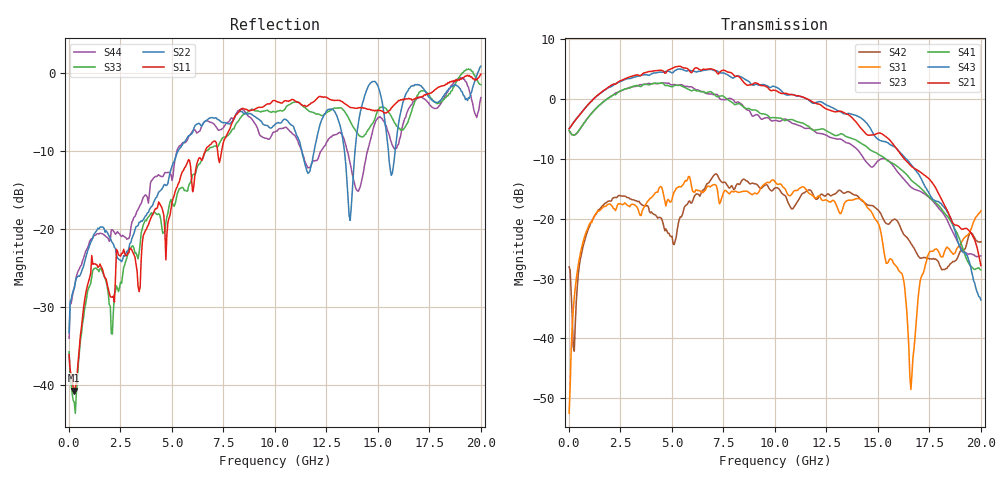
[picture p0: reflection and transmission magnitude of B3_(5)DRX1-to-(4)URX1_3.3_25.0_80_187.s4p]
!Agilent Technologies,N5225A,MY51451112,A.09.50.13
!Agilent N5225A: A.09.50.13
!Date: Sunday, March 12, 2017 05:22:41
!Correction: S11(Full 4 Port(1,2,3,4))
!S12(Full 4 Port(1,2,3,4))
!S13(Full 4 Port(1,2,3,4))
!S14(Full 4 Port(1,2,3,4))
!S21(Full 4 Port(1,2,3,4))
!S22(Full 4 Port(1,2,3,4))
!S23(Full 4 Port(1,2,3,4))
!S24(Full 4 Port(1,2,3,4))
!S31(Full 4 Port(1,2,3,4))
!S32(Full 4 Port(1,2,3,4))
!S33(Full 4 Port(1,2,3,4))
!S34(Full 4 Port(1,2,3,4))
!S41(Full 4 Port(1,2,3,4))
!S42(Full 4 Port(1,2,3,4))
!S43(Full 4 Port(1,2,3,4))
!S44(Full 4 Port(1,2,3,4))
!S4P File: Measurements: <S11,S12,S13,S14>,
!<S21,S22,S23,S24>,
!<S31,S32,S33,S34>,
!<S41,S42,S43,S44>:
# Hz S  dB  R 50
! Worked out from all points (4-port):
!   401 points, 10 MHz to 20 GHz, reference 50 ohm
!   strongest paths, dB at 10 MHz, 5.008 GHz, 10.01 GHz, 15 GHz, 20 GHz:
!     S21: -5.0, 5.1, 1.4, -5.8, -27.8
!     S43: -5.0, 4.3, 2.0, -6.7, -33.6
!     S41: -5.3, 2.0, -3.2, -9.2, -28.6
!     S23: -5.3, 2.3, -3.6, -10.4, -26.2
!     S31: -52.5, -16.8, -13.9, -20.7, -18.7
!     S42: -28.0, -23.0, -14.9, -18.5, -23.9
!   lowest |S11| = -40.8 dB at 259.9 MHz (marker M1), VSWR 1.02, Z = 50.3 - j0.878 ohm
!   |S11| at or under -10 dB: start of sweep to 6.627 GHz; 7.217 GHz to 7.417 GHz (199.7 MHz wide, 2.73 % of centre)
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1e7  -36.13 -37.8  -63.03 122.5  -53.14 14.6  -71.38 138.6
     -5.01 1.8  -33.32 39.3  -5.33 -179.5  -27.99 38.1
     -52.49 14.4  -64.49 116.4  -35.78 -47.0  -64.85 112.1
     -5.33 -179.5  -28.05 37.1  -5.00 2.0  -34.03 44.9
2.59875e8  -40.75 -72.3  -49.94 54.9  -33.10 94.8  -50.18 53.7
           -3.81 4.3  -27.60 -131.8  -6.08 178.3  -41.85 -162.0
           -33.19 95.1  -49.91 56.7  -42.27 -78.7  -50.38 55.0
           -6.08 177.5  -42.12 -170.9  -3.80 3.5  -27.66 -137.8
2.958525e9  -22.49 148.5  -43.03 -34.4  -17.68 52.3  -42.63 -60.4
            3.65 -93.6  -21.90 160.4  1.88 78.3  -16.75 38.8
            -18.04 54.6  -42.45 -31.0  -22.54 117.8  -41.33 -56.5
            1.76 68.8  -16.73 39.3  3.34 -101.3  -20.91 145.2
5.057475e9  -16.12 90.7  -41.14 10.6  -15.98 28.2  -39.26 -28.8
            5.15 170.8  -11.58 146.6  2.33 -25.4  -24.36 44.4
            -16.03 28.2  -37.69 -2.7  -16.93 102.4  -33.27 -40.9
            2.04 -40.4  -24.21 41.5  4.36 160.1  -13.17 126.5
8.2059e9  -5.16 36.4  -38.89 -114.7  -15.70 2.0  -36.78 -142.3
          3.74 14.5  -5.06 82.0  -0.55 -172.7  -13.86 47.3
          -15.61 1.2  -32.78 -112.9  -6.26 58.9  -31.99 -145.1
          -0.86 164.1  -14.17 51.4  3.79 1.7  -4.88 46.1
1.155422e10  -4.28 -6.2  -37.43 -117.8  -14.86 -22.4  -40.10 -136.5
             -0.02 -130.4  -12.60 85.5  -4.95 45.2  -15.34 37.1
             -15.36 -23.6  -33.59 -123.1  -4.71 10.4  -34.14 -151.9
             -4.48 7.1  -15.38 42.2  -0.05 -155.5  -11.90 25.4
2e10  -0.18 -114.1  -32.92 62.6  -18.73 121.3  -35.50 21.8
      -27.84 -160.3  0.84 17.1  -26.22 23.3  -23.90 101.9
      -18.70 121.3  -34.00 40.1  -1.53 -87.7  -35.27 -7.8
      -28.56 -24.2  -23.88 102.7  -33.58 170.5  -3.18 -136.6
